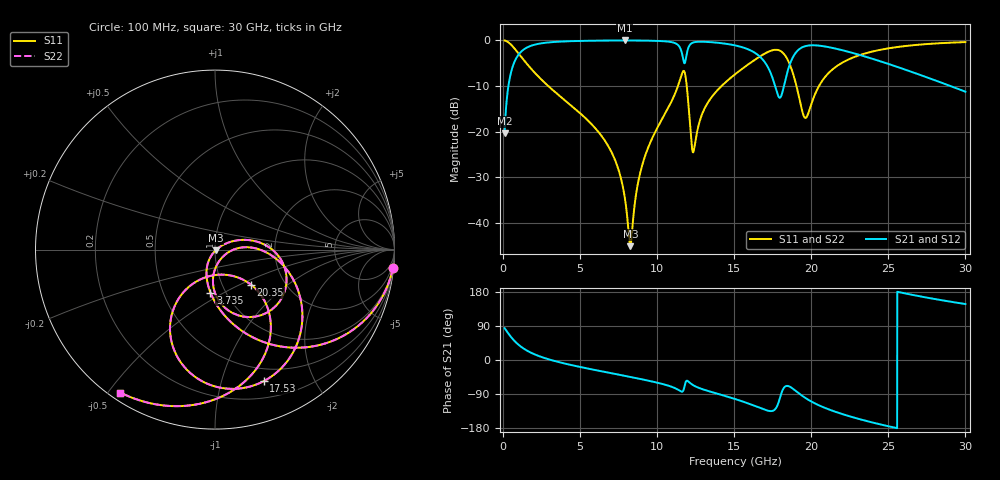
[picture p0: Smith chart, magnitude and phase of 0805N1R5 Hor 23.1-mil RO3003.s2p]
# GHz S MA R 50
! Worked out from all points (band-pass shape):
!   3201 points, 100 MHz to 30 GHz, reference 50 ohm
!   highest |S21| = -0.05 dB at 7.893 GHz (marker M1); lowest = -20.4 dB at 100 MHz (marker M2)
!   |S21| within 3 dB of the highest: 1.026 GHz to 11.62 GHz (10.6 GHz wide, 168 % of centre); 11.92 GHz to 16.47 GHz (4.557 GHz wide, 32.1 % of centre)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
!   lowest |S11| = -45.1 dB at 8.257 GHz (marker M3), VSWR 1.01, Z = 50.4 - j0.402 ohm
!   |S11| at or under -10 dB: 2.926 GHz to 11.35 GHz (8.423 GHz wide, 118 % of centre); 11.92 GHz to 14.18 GHz (2.266 GHz wide, 17.4 % of centre); 19.04 GHz to 20.5 GHz (1.467 GHz wide, 7.42 % of centre)
!   |S22| runs from -45.1 to 0.0 dB; largest |S21 - S12| = 0
!   S11 on the Smith chart (normalised r, x): 100 MHz: 1, -19; 3.735 GHz: 0.85, -0.43; 17.53 GHz: 0.36, -1.37; 20.35 GHz: 1.36, -0.58; 30 GHz: 0.03, -0.54
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0.1  0.9954 -6.0  0.09567 83.9  0.09567 83.9  0.9954 -6.0
0.9689688  0.7293 -48.5  0.6831 41.4  0.6831 41.4  0.7293 -48.5
3.734719  0.2408 -96.0  0.9676 -6.7  0.9676 -6.7  0.2408 -96.0
5.089563  0.154 -107.8  0.9844 -19.1  0.9844 -19.1  0.154 -107.8
6.977  0.06232 -120.3  0.9933 -34.5  0.9933 -34.5  0.06232 -120.3
7.892688  0.01921 -116.0  0.9943 -41.8  0.9943 -41.8  0.01921 -116.0
8.257094  0.005557 -45.9  0.9941 -44.7  0.9941 -44.7  0.005557 -45.9
8.939187  0.03763 29.9  0.9926 -50.3  0.9926 -50.3  0.03763 29.9
10.06978  0.1148 24.7  0.9835 -60.5  0.9835 -60.5  0.1148 24.7
11.25644  0.2864 4.6  0.9132 -76.3  0.9132 -76.3  0.2864 4.6
11.70494  0.4616 -38.7  0.6041 -79.6  0.6041 -79.6  0.4616 -38.7
12.36834  0.06103 -31.8  0.9492 -67.3  0.9492 -67.3  0.06103 -31.8
13.20928  0.1971 3.5  0.9599 -80.6  0.9599 -80.6  0.1971 3.5
15.05  0.4238 -16.5  0.8793 -102.9  0.8793 -102.9  0.4238 -16.5
17.52609  0.7816 -69.6  0.3688 -133.7  0.3688 -133.7  0.7816 -69.6
17.99328  0.7645 -89.4  0.2362 -96.4  0.2362 -96.4  0.7645 -89.4
18.638  0.5265 -118.3  0.5639 -71.2  0.5639 -71.2  0.5265 -118.3
19.535  0.1453 -96.4  0.8541 -98.0  0.8541 -98.0  0.1453 -96.4
20.03956  0.208 -49.5  0.8815 -110.4  0.8815 -110.4  0.208 -49.5
20.34791  0.281 -44.2  0.8784 -116.8  0.8784 -116.8  0.281 -44.2
25.01978  0.8165 -86.9  0.5497 -175.0  0.5497 -175.0  0.8165 -86.9
30  0.9553 -123.5  0.2735 147.7  0.2735 147.7  0.9553 -123.5
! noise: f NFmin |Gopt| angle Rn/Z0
0.1  0.001003  0.9437  1.672  0.003986
3.417  0.007357  0.741  19.64  0.005531
6.743  0.01293  0.7182  37.05  0.008183
10.06  0.02294  0.7637  53.65  0.01577
13.39  0.03748  0.8087  69.81  0.0276
16.7  0.11  0.9165  85.15  0.1578
20.03  0.1063  0.8996  99.78  0.09649
23.35  0.07519  0.8435  112.7  0.03183
26.67  0.08311  0.8438  125  0.0247
30  0.1047  0.8652  137.2  0.02301
